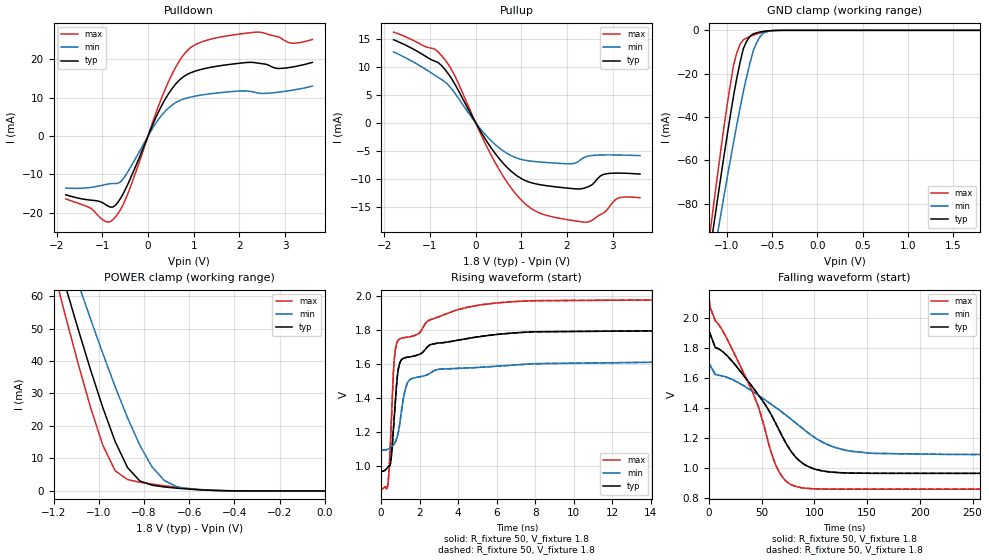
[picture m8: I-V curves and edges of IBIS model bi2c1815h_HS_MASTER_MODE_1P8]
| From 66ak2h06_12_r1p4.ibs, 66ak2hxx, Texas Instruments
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|   Model Cell bi2c1815h_HS_MASTER_MODE_1P8
|bi2c1815h_HS_MASTER_MODE_1P8
[Model]   bi2c1815h_HS_MASTER_MODE_1P8
Model_type   I/O
Polarity   Non-Inverting
Enable   Active-Low
Vinl =  0.54
Vinh =  1.26
Cref =  15.0000pF
Rref =  100.0000M
Vref =  0V
Vmeas =  0.9
C_comp   7.82904p   2.84791p   8.43627p
[Model Spec]
Vinl   0.54   0.486   0.594
Vinh   1.26   1.134   1.386
[Temperature Range]   25   125   -40
[Voltage Range]   1.8   1.62   1.98
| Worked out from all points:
|   slope of the pulldown table from 0 to 0.27 V, typ, clamps not added: 37.1 ohm
|   slope of the pullup table from 0 to 0.27 V, typ, clamps not added: 73.7 ohm
|   GND clamp passes 1 mA (typ) near -0.66 V on its own axis
|   POWER clamp passes 1 mA (typ) near -0.68 V on its own axis
|   rising waveform, R_fixture 50, V_fixture 1.8: 20-80 % time 596ps typ, 749ps min, 963ps max; typ from 0.966 V to 1.8 V
|   rising waveform, R_fixture 50, V_fixture 1.8: 20-80 % time 596ps typ, 749ps min, 963ps max; typ from 0.966 V to 1.8 V
|   falling waveform, R_fixture 50, V_fixture 1.8: 20-80 % time 44.9ns typ, 60.9ns min, 35.5ns max; typ from 1.8 V to 0.966 V
|   falling waveform, R_fixture 50, V_fixture 1.8: 20-80 % time 44.9ns typ, 60.9ns min, 35.5ns max; typ from 1.8 V to 0.966 V
| Nom Voltages:
|   VDD=0.95, VDDS=1.8, ESD_BIASFET=0, VSS=0, VSSS=0
| Min Voltages:
|   VDD=0.81, VDDS=1.62, ESD_BIASFET=0, VSS=0, VSSS=0
| Max Voltages:
|   VDD=0.998, VDDS=1.98, ESD_BIASFET=0, VSS=0, VSSS=0
[POWER_clamp]
|   voltage   I(typ)   I(min)   I(max)
-1.8V     228.3mA    217.1mA    239.9mA
-1.182V   71.41mA    82.7mA     63.22mA
-1.164V   67.02mA    78.9mA     58.31mA
-1.127V   58.34mA    71.38mA    48.65mA
-1.073V   45.63mA    60.27mA    34.69mA
-981.8mV  25.64mA    42.31mA    14.07mA
-927.3mV  15.19mA    32.09mA    6.201mA
-872.7mV  7.212mA    22.55mA    3.494mA
-818.2mV  3.071mA    14.07mA    2.668mA
-763.6mV  1.749mA    7.355mA    2.087mA
-654.5mV  846uA      1.319mA    1.117mA
0V        320pA      6.203nA    1.2nA
[Pulldown]
|   voltage   I(typ)   I(min)   I(max)
-1.8V     -15.34mA   -13.56mA   -16.43mA
-1.255V   -16.73mA   -13.41mA   -18.86mA
-927.3mV  -17.92mA   -12.65mA   -22.3mA
-709.1mV  -18.01mA   -12.41mA   -21.06mA
-436.4mV  -12.4mA    -9.209mA   -14.87mA
109.1mV   3.162mA    2.233mA    3.875mA
381.8mV   9.743mA    6.546mA    12.41mA
709.1mV   14.85mA    9.354mA    20.03mA
981.8mV   16.74mA    10.31mA    23.49mA
2.345V    19.16mA    11.4mA     27.11mA
3.164V    18.03mA    11.98mA    24.23mA
3.6V      19.24mA    13.03mA    25.22mA
[Pullup]
|   voltage   I(typ)   I(min)   I(max)
-1.8V     14.85mA    12.68mA    16.22mA
-927.3mV  11.12mA    8.671mA    13.28mA
-654.5mV  9.345mA    7.19mA     11.08mA
-436.4mV  6.627mA    5.079mA    8.046mA
436.4mV   -5.591mA   -3.953mA   -7.27mA
818.2mV   -8.949mA   -6.033mA   -12.12mA
1.2V      -10.68mA   -6.846mA   -15.24mA
2.127V    -11.78mA   -7.31mA    -17.49mA
2.455V    -11.46mA   -5.985mA   -17.76mA
2.782V    -9.301mA   -5.75mA    -16.22mA
3.109V    -9mA       -5.76mA    -13.52mA
3.6V      -9.17mA    -5.88mA    -13.41mA
[GND_clamp]
|   voltage   I(typ)   I(min)   I(max)
-1.8V     -287mA     -272.2mA   -302.8mA
-1.182V   -100.5mA   -113.1mA   -91.98mA
-1.145V   -89.92mA   -104mA     -80.05mA
-1.109V   -79.52mA   -95.11mA   -68.4mA
-1.073V   -69.22mA   -86.23mA   -56.94mA
-927.3mV  -30.39mA   -51.8mA    -16.31mA
-890.9mV  -22.12mA   -43.71mA   -10.41mA
-818.2mV  -8.424mA   -28.23mA   -4.346mA
-709.1mV  -1.635mA   -9.541mA   -2.241mA
-600mV    -499.1uA   -1.337mA   -852.9uA
-490.9mV  -80.16uA   -133.6uA   -148.6uA
1.8V      320.1pA    340nA      252.2pA
[Ramp]
| variable   typ   min   max
dV/dt_f   0.562728/52.675392n   0.3582/71.070158n   0.757608/42.33264n
dV/dt_r   0.40035/38.001848n  0.2579736/59.625943n   0.554496/27.238686n
R_load = 50
[Rising Waveform]
R_fixture = 50
V_fixture = 1.8
V_fixture_min = 1.62
V_fixture_max = 1.98
|   time   V(typ)   V(min)   V(max)
0s        966.2mV    1.092V     862.2mV
358.2ps   993.4mV    1.097V     899.7mV
509.7ps   1.033V     1.106V     1.213V
669ps     1.271V     1.125V     1.61V
886.6ps   1.566V     1.194V     1.738V
1.238ns   1.635V     1.442V     1.754V
1.563ns   1.642V     1.511V     1.76V
4.016ns   1.739V     1.572V     1.919V
7.908ns   1.788V     1.6V       1.97V
1.25us    1.8V       1.62V      1.98V
[Rising Waveform]
R_fixture = 50
V_fixture = 1.8
V_fixture_min = 1.62
V_fixture_max = 1.98
|   time   V(typ)   V(min)   V(max)
0s        966.2mV    1.092V     862.2mV
358.2ps   993.4mV    1.097V     899.7mV
509.7ps   1.033V     1.106V     1.213V
669ps     1.271V     1.125V     1.61V
886.6ps   1.566V     1.194V     1.738V
1.238ns   1.635V     1.442V     1.754V
1.563ns   1.642V     1.511V     1.76V
4.016ns   1.739V     1.572V     1.919V
7.908ns   1.788V     1.6V       1.97V
1.25us    1.8V       1.62V      1.98V
[Falling Waveform]
R_fixture = 50
V_fixture = 1.8
V_fixture_min = 1.62
V_fixture_max = 1.98
|   time   V(typ)   V(min)   V(max)
0s        1.8V       1.62V      1.98V
346.5ps   1.896V     1.636V     2.124V
865.9ps   1.899V     1.689V     2.077V
6.116ns   1.802V     1.622V     1.98V
40.68ns   1.547V     1.515V     1.519V
67.37ns   1.242V     1.384V     966.2mV
90.39ns   1.026V     1.256V     868.2mV
118.5ns   973.1mV    1.14V      861.6mV
155.4ns   966.6mV    1.099V     861.3mV
1.25us    966.2mV    1.092V     861.3mV
[Falling Waveform]
R_fixture = 50
V_fixture = 1.8
V_fixture_min = 1.62
V_fixture_max = 1.98
|   time   V(typ)   V(min)   V(max)
0s        1.8V       1.62V      1.98V
346.5ps   1.896V     1.636V     2.124V
865.9ps   1.899V     1.689V     2.077V
6.116ns   1.802V     1.622V     1.98V
40.68ns   1.547V     1.515V     1.519V
67.37ns   1.242V     1.384V     966.2mV
90.39ns   1.026V     1.256V     868.2mV
118.5ns   973.1mV    1.14V      861.6mV
155.4ns   966.6mV    1.099V     861.3mV
1.25us    966.2mV    1.092V     861.3mV
